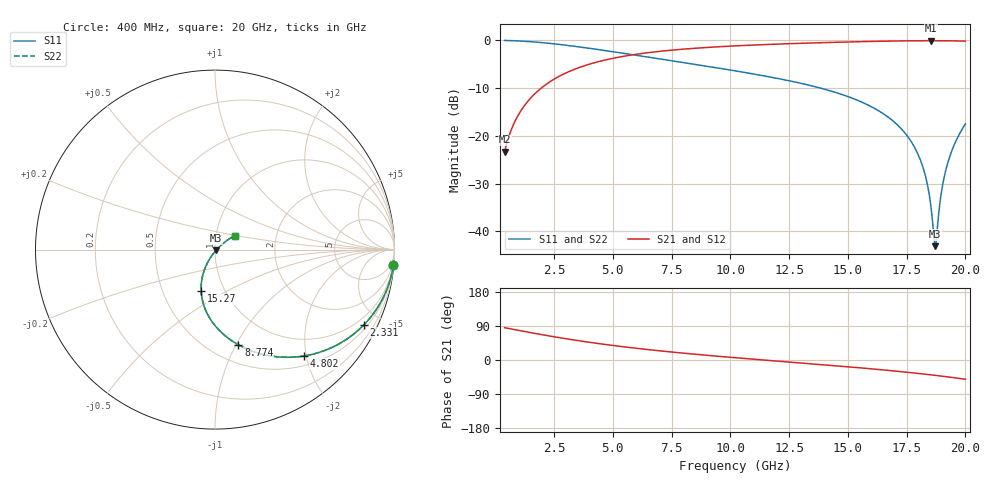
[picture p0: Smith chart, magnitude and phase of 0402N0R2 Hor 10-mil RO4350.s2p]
# GHz S MA R 50
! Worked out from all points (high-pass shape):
!   1960 points, 400 MHz to 20 GHz, reference 50 ohm
!   highest |S21| = -0.07 dB at 18.55 GHz (marker M1); lowest = -23.3 dB at 400 MHz (marker M2)
!   |S21| within 3 dB of the highest: 5.796 GHz to end of sweep
!   lowest |S11| = -43.1 dB at 18.72 GHz (marker M3), VSWR 1.01, Z = 50.5 - j0.463 ohm
!   |S11| at or under -10 dB: 13.84 GHz to end of sweep
!   |S22| runs from -43.1 to 0.0 dB; largest |S21 - S12| = 0
!   S11 on the Smith chart (normalised r, x): 400 MHz: 1, -24; 2.331 GHz: 0.66, -4.09; 4.802 GHz: 0.67, -1.96; 8.774 GHz: 0.68, -1.02; 15.27 GHz: 0.78, -0.38; 20 GHz: 1.23, +0.19
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0.4  0.9977 -4.8  0.068 85.2  0.068 85.2  0.9977 -4.8
1.140378  0.9816 -13.5  0.1907 76.4  0.1907 76.4  0.9816 -13.5
2.330985  0.9293 -26.9  0.3689 63.1  0.3689 63.1  0.9293 -26.9
3.671669  0.8476 -40.2  0.5298 49.8  0.5298 49.8  0.8476 -40.2
4.802246  0.7736 -50.0  0.6327 40.0  0.6327 40.0  0.7736 -50.0
6.943338  0.6426 -65.4  0.7647 24.5  0.7647 24.5  0.6426 -65.4
8.774273  0.5465 -76.2  0.8356 13.7  0.8356 13.7  0.5465 -76.2
10.205  0.4794 -83.7  0.8754 6.1  0.8754 6.1  0.4794 -83.7
13.46667  0.3336 -99.6  0.9393 -10.1  0.9393 -10.1  0.3336 -99.6
15.26759  0.2436 -108.4  0.9655 -19.3  0.9655 -19.3  0.2436 -108.4
16.73834  0.1555 -115.7  0.9823 -27.5  0.9823 -27.5  0.1555 -115.7
17.4487  0.1056 -118.9  0.9882 -31.9  0.9882 -31.9  0.1056 -118.9
17.96896  0.06538 -120.0  0.9911 -35.3  0.9911 -35.3  0.06538 -120.0
18.31914  0.03638 -117.4  0.9921 -37.7  0.9921 -37.7  0.03638 -117.4
18.54926  0.01696 -105.8  0.9924 -39.3  0.9924 -39.3  0.01696 -105.8
18.65932  0.008874 -79.0  0.9923 -40.1  0.9923 -40.1  0.008874 -79.0
18.71935  0.006986 -41.0  0.9922 -40.5  0.9922 -40.5  0.006986 -41.0
18.77938  0.008977 -2.9  0.9921 -41.0  0.9921 -41.0  0.008977 -2.9
18.98948  0.0266 31.4  0.9915 -42.6  0.9915 -42.6  0.0266 31.4
19.19959  0.04697 36.4  0.9905 -44.2  0.9905 -44.2  0.04697 36.4
19.54977  0.08314 37.3  0.9875 -47.0  0.9875 -47.0  0.08314 37.3
20  0.1332 35.3  0.9813 -50.8  0.9813 -50.8  0.1332 35.3
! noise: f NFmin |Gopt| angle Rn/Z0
0.4  0.002398  0.9343  4.504  0.00812
2.571  0.004361  0.7014  16.37  0.002805
4.752  0.00648  0.6057  20.89  0.002944
6.933  0.008653  0.5615  24.31  0.003403
9.104  0.01099  0.5427  27.43  0.00405
11.29  0.01366  0.5406  30.43  0.004944
13.47  0.01688  0.5519  33.35  0.006221
15.64  0.02093  0.5753  36.25  0.008139
17.82  0.02643  0.6111  39.25  0.01126
20  0.03442  0.6592  42.45  0.01687
